FUNCTION_BLOCK FB_LN_IED_LD1_LEDGGIO6 EXTENDS FB_AcsiCommonLogicalNodeClass
VAR_INPUT
	NamPlt: FB_DO_IED_LD1_LEDGGIO6_NamPlt := (sClass:='LPL', bLinkResult:=THIS^.AddDataToContainer(ipData:=NamPlt));
	Beh: FB_DO_IED_LD1_LEDGGIO6_Beh := (sClass:='ENS', bLinkResult:=THIS^.AddDataToContainer(ipData:=Beh));
	Health: FB_DO_IED_LD1_LEDGGIO6_Health := (sClass:='ENS', bLinkResult:=THIS^.AddDataToContainer(ipData:=Health));
	Mod_: FB_DO_IED_LD1_LEDGGIO6_Mod := (sObjectName:='Mod', sClass:='ENC', bLinkResult:=THIS^.AddDataToContainer(ipData:=Mod_));
	AnOut1: FB_DO_IED_LD1_LEDGGIO6_AnOut1 := (sClass:='APC', bLinkResult:=THIS^.AddDataToContainer(ipData:=AnOut1));
	SPCSO1: FB_DO_IED_LD1_LEDGGIO6_SPCSO1 := (sClass:='SPC', bLinkResult:=THIS^.AddDataToContainer(ipData:=SPCSO1));
	DPCSO1: FB_DO_IED_LD1_LEDGGIO6_DPCSO1 := (sClass:='DPC', bLinkResult:=THIS^.AddDataToContainer(ipData:=DPCSO1));
	ISCSO1: FB_DO_IED_LD1_LEDGGIO6_ISCSO1 := (sClass:='INC', bLinkResult:=THIS^.AddDataToContainer(ipData:=ISCSO1));
END_VAR
VAR
END_VAR

END_FUNCTION_BLOCK
